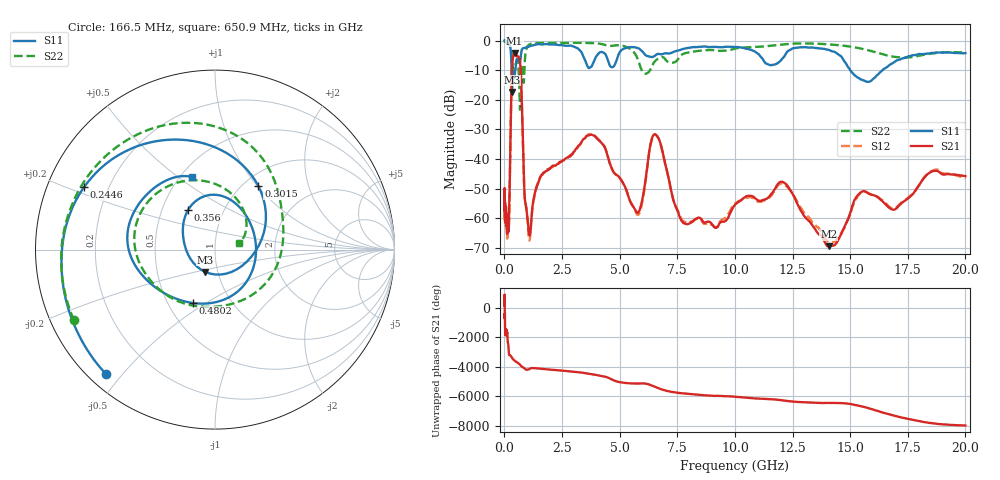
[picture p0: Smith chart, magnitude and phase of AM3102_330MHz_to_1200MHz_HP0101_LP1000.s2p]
! Date/Time: Tue, Sep 11, 2018 5:14 PM
! Network Analyzer: Agilent Technologies E8362B Rev: A.07.50.63
! Sweep from 0.010 to 20.000 GHz, 1601 Points, Sweep Type: LOG
! Power Supply: 4.949 V, 0.001 A
# Hz S DB R 50
!freq MagS11 AngS11 MagS21 AngS21 MagS12 AngS12 MagS22 AngS22
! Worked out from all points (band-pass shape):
!   1601 points, 10 MHz to 20 GHz, reference 50 ohm
!   highest |S21| = -4.23 dB at 445.1 MHz (marker M1); lowest = -69.4 dB at 14.07 GHz (marker M2)
!   |S21| within 3 dB of the highest: 345.9 MHz to 678.4 MHz (332.5 MHz wide, 64.9 % of centre)
!   lowest |S11| = -17.4 dB at 331.5 MHz (marker M3), VSWR 1.31, Z = 43.6 - j11 ohm
!   |S11| at or under -10 dB: 309.7 MHz to 477.8 MHz (168.1 MHz wide, 42.7 % of centre); 15.01 GHz to 16.41 GHz (1.4 GHz wide, 8.91 % of centre)
!   |S22| runs from -23.4 to -0.3 dB; largest |S21 - S12| = 0.012
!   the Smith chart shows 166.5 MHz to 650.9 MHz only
!   S11 on the Smith chart (normalised r, x): 166.5 MHz: 0.05, -0.45; 244.6 MHz: 0.11, +0.23; 301.5 MHz: 1.17, +1.01; 356 MHz: 0.68, +0.32; 480.2 MHz: 0.66, -0.44; 650.9 MHz: 0.57, +0.56
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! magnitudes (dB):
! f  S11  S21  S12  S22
! 10 MHz  0.0  -50.7  -50.3  -0.3
! 35.55 MHz  0.0  -58.2  -60.0  -0.5
! 126.4 MHz  -0.4  -64.0  -66.4  -0.9
! 166.5 MHz  -0.7  -63.6  -63.5  -1.1
! 244.6 MHz  -1.9  -43.0  -43.0  -1.8
! 301.5 MHz  -7.4  -17.4  -17.4  -3.7
! 331.5 MHz  -17.4  -9.0  -9.0  -6.6
! 356 MHz  -11.5  -6.5  -6.6  -8.4
! 445.1 MHz  -11.8  -4.2  -4.3  -9.2
! 447.2 MHz  -11.7  -4.2  -4.3  -9.1
! 480.2 MHz  -9.8  -4.3  -4.4  -8.1
! 650.9 MHz  -7.4  -6.0  -6.1  -17.0
! 873.8 MHz  -2.4  -52.0  -52.2  -9.3
! 1.072 GHz  -2.0  -65.0  -67.2  -1.4
! 1.59 GHz  -1.3  -45.6  -45.7  -0.8
! 3.793 GHz  -8.6  -31.8  -31.7  -0.8
! 5.652 GHz  -2.3  -56.9  -57.2  -4.3
! 6.58 GHz  -4.8  -31.8  -32.0  -6.6
! 7.845 GHz  -2.7  -61.8  -61.4  -4.3
! 12.09 GHz  -5.9  -47.8  -48.3  -1.3
! 14.07 GHz  -3.2  -69.4  -68.0  -1.3
! 20 GHz  -4.3  -45.8  -46.5  -4.0
